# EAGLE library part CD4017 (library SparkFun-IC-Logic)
10-Out Decade Counter Datasheet SparkFun Products SparkFun SparkPunk Sequencer Kit (KIT-12707)
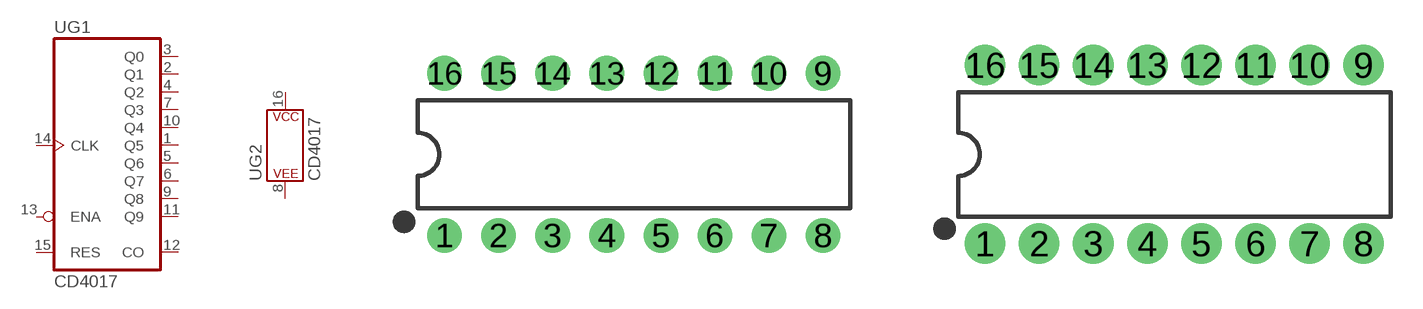
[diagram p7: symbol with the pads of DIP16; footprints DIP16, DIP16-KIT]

Designator prefix U; gates G1=CD4017 G2=POWER_CONSORT

## CD4017 (PROD_ID: IC-11929; VALUE: CD4017)  [DIP16]
1  G1:Q5  out
2  G1:Q1  out
3  G1:Q0  out
4  G1:Q2  out
5  G1:Q6  out
6  G1:Q7  out
7  G1:Q3  out
8  G2:P$V-
9  G1:Q8  out
10  G1:Q4  out
11  G1:Q9  out
12  G1:CO  out
13  G1:ENA  in
14  G1:CLK  in
15  G1:RES  in
16  G2:P$V+

## CD4017KIT (PROD_ID: IC-11929)  [DIP16-KIT]
Pads as for DIP16

## Footprint DIP16 (pad centres in mm)
Dual In Line Package
drill 0.813 pad 1.626: 1 -8.89,-3.81; 2 -6.35,-3.81; 3 -3.81,-3.81; 4 -1.27,-3.81; 5 1.27,-3.81; 6 3.81,-3.81; 7 6.35,-3.81; 8 8.89,-3.81; 9 8.89,3.81; 10 6.35,3.81; 11 3.81,3.81; 12 1.27,3.81; 13 -1.27,3.81; 14 -3.81,3.81; 15 -6.35,3.81; 16 -8.89,3.81

## Footprint DIP16-KIT (pad centres in mm)
drill 0.864 pad 1.905: 1 -8.89,-4.191; 2 -6.35,-4.191; 3 -3.81,-4.191; 4 -1.27,-4.191; 5 1.27,-4.191; 6 3.81,-4.191; 7 6.35,-4.191; 8 8.89,-4.191; 9 8.89,4.191; 10 6.35,4.191; 11 3.81,4.191; 12 1.27,4.191; 13 -1.27,4.191; 14 -3.81,4.191; 15 -6.35,4.191; 16 -8.89,4.191

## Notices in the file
Licensing: Creative Commons ShareAlike 4.0 International - https://creativecommons.org/licenses/by-sa/4.0
